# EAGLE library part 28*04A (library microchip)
CMOS EPROM 4 K (512 x 8) Source: ww1.microchip.com/downloads/en/DeviceDoc/11126H.pdf
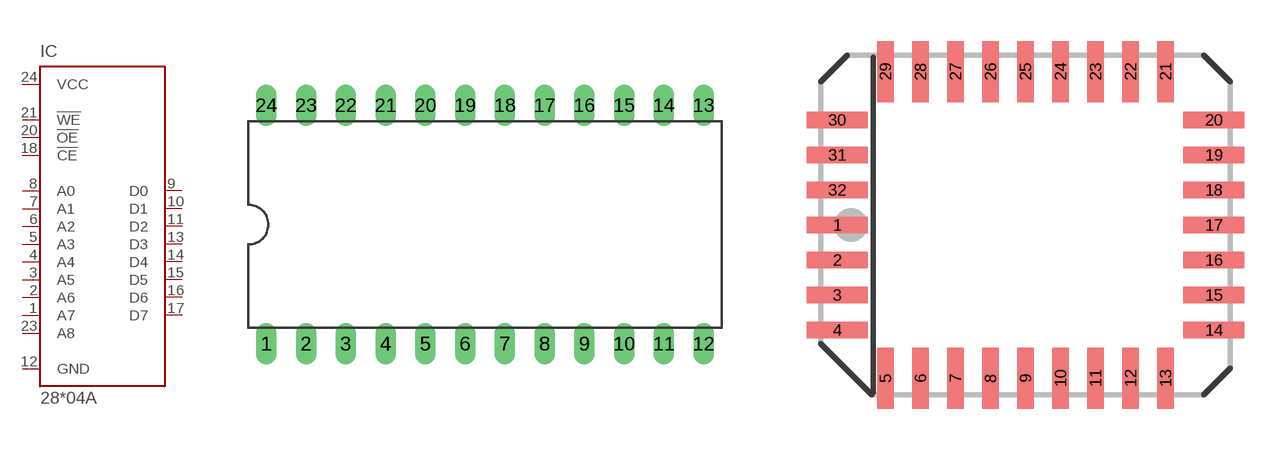
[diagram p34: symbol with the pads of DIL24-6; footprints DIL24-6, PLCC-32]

Designator prefix IC

## 28C04AP (OC_FARNELL: unknown; OC_NEWARK: unknown)  [DIL24-6]
1  A7  in
2  A6  in
3  A5  in
4  A4  in
5  A3  in
6  A2  in
7  A1  in
8  A0  in
9  D0  hiz
10  D1  hiz
11  D2  hiz
12  GND  pwr
13  D3  hiz
14  D4  hiz
15  D5  hiz
16  D6  hiz
17  D7  hiz
18  !CE  in
19  NC19  nc
20  !OE  in
21  !WE  in
22  NC22  nc
23  A8  in
24  VCC  pwr

## 28C04AL (OC_FARNELL: unknown; OC_NEWARK: unknown)  [PLCC-32]
1  NC19  nc
4  A7  in
5  A6  in
6  A5  in
7  A4  in
8  A3  in
9  A2  in
10  A1  in
11  A0  in
13  D0  hiz
14  D1  hiz
15  D2  hiz
16  GND  pwr
17  NC22  nc
18  D3  hiz
19  D4  hiz
20  D5  hiz
21  D6  hiz
22  D7  hiz
23  !CE  in
25  !OE  in
29  A8  in
31  !WE  in
32  VCC  pwr

## Footprint DIL24-6 (pad centres in mm)
Dual In Line package type P
drill 0.813 long: 1 -13.97,-7.62; 2 -11.43,-7.62; 3 -8.89,-7.62; 4 -6.35,-7.62; 5 -3.81,-7.62; 6 -1.27,-7.62; 7 1.27,-7.62; 8 3.81,-7.62; 9 6.35,-7.62; 10 8.89,-7.62; 11 11.43,-7.62; 12 13.97,-7.62; 13 13.97,7.62; 14 11.43,7.62; 15 8.89,7.62; 16 6.35,7.62; 17 3.81,7.62; 18 1.27,7.62; 19 -1.27,7.62; 20 -3.81,7.62; 21 -6.35,7.62; 22 -8.89,7.62; 23 -11.43,7.62; 24 -13.97,7.62

## Footprint PLCC-32 (pad centres in mm)
PLASTIC LEADED CHIP CARRIER rectangle, package type L
smd 2.2 x 0.6: 1 -6.83,0; 2 -6.83,-1.27; 3 -6.83,-2.54; 4 -6.83,-3.81; 14 6.83,-3.81; 15 6.83,-2.54; 16 6.83,-1.27; 17 6.83,0; 18 6.83,1.27; 19 6.83,2.54; 20 6.83,3.81; 30 -6.83,3.81; 31 -6.83,2.54; 32 -6.83,1.27
smd 0.6 x 2.2: 5 -5.08,-5.56; 6 -3.81,-5.56; 7 -2.54,-5.56; 8 -1.27,-5.56; 9 0,-5.56; 10 1.27,-5.56; 11 2.54,-5.56; 12 3.81,-5.56; 13 5.08,-5.56; 21 5.08,5.56; 22 3.81,5.56; 23 2.54,5.56; 24 1.27,5.56; 25 0,5.56; 26 -1.27,5.56; 27 -2.54,5.56; 28 -3.81,5.56; 29 -5.08,5.56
